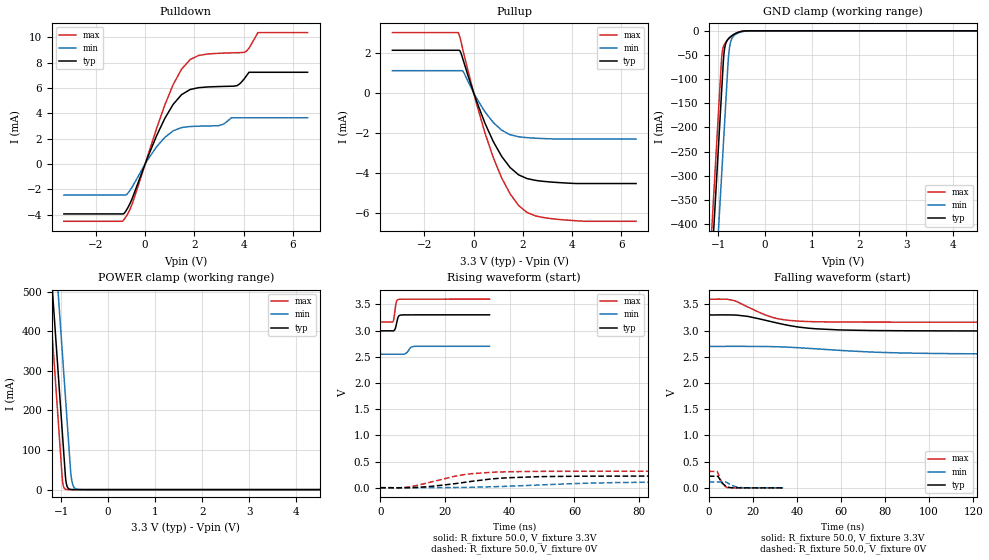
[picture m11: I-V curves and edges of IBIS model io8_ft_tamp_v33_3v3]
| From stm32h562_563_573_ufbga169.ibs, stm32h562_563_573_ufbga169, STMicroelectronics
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[Model]   io8_ft_tamp_v33_3v3
Model_type I/O
Polarity   Non-Inverting
Enable   Active-Low
| CAP_THRESHOLD on pad IOFT is "UDTCAPC" :
| Rising=20.0% of vddiom   Falling=80.0% of vddiom
| C_comp min and max val. don't necessarily correlate with the min and max pvt
| but are the smallest and greatest pad capacitance found.
| var   typ   min   max
C_comp   8.23612pF  8.16297pF  8.41737pF
|C_comp_pullup   5.18195pF  4.95450pF  4.90580pF
|C_comp_pulldown   3.05417pF  3.20847pF  3.51157pF
Vinl = 1.35V
Vinh = 1.8V
Vmeas = 1.65V   | Reference voltage for timing measurements
Cref  = 50.0pF   | Timing specification test load capacitance value
Rref  = 1.0MOhm   | Timing specification test load resistance value
Vref  = 1.815V   | Timing specification test load voltage
[Model Spec]
| TIME_THRESHOLD on pin ZIV33SW is "CMOS" :
| Rising=40.0% of VDDV33SW   Falling=60.0% of VDDV33SW
Vinl 1.28980V 1.06780V 1.39680V
Vinh 1.76120V 1.48020V 1.88320V
| variable   typ   min   max
[Temperature Range] 25.0 125.0 -40.0
| variable   typ   min   max
[Voltage Range] 3.3V 2.7V 3.6V
| variable   typ   min   max
[POWER Clamp Reference] 3.3V 2.7V 3.6V
| variable   typ   min   max
[GND Clamp Reference] 0V 0V 0V
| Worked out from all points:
|   slope of the pulldown table from 0 to 0.495 V, typ, clamps not added: 211 ohm
|   slope of the pullup table from 0 to 0.495 V, typ, clamps not added: 307 ohm
|   GND clamp passes 1 mA (typ) near -0.49 V on its own axis
|   POWER clamp passes 1 mA (typ) near -0.82 V on its own axis
|   rising waveform, R_fixture 50.0, V_fixture 3.3V: 20-80 % time 707ps typ, 1.09ns min, 576ps max; typ from 2.99 V to 3.3 V
|   falling waveform, R_fixture 50.0, V_fixture 3.3V: 20-80 % time 22.1ns typ, 40.6ns min, 14.5ns max; typ from 3.3 V to 2.99 V
|   rising waveform, R_fixture 50.0, V_fixture 0V: 20-80 % time 17.9ns typ, 30.6ns min, 13.5ns max; typ from 0 V to 0.222 V
|   falling waveform, R_fixture 50.0, V_fixture 0V: 20-80 % time 2.6ns typ, 3.54ns min, 2.19ns max; typ from 0.222 V to 0 V
[POWER Clamp]
-3.3V     4.099A     4.3A       3.98A
-1.25V    613.6mA    815.2mA    494.9mA
-1.17V    477.6mA    679.2mA    358.9mA
-1.13V    409.6mA    611.2mA    290.9mA
-1.02V    222.6mA    424.2mA    103.9mA
-970mV    137.6mA    339.2mA    21.83mA
-910mV    35.64mA    237.2mA    1.102mA
-870mV    7.512mA    169.2mA    150.4uA
-790mV    333.8uA    37.52mA    2.807uA
-750mV    70.36uA    11.69mA    384.4nA
-670mV    3.13uA     1.135mA    8.16nA
6.6V      0A         0A         0A
[GND Clamp]
-3.3V     -4.162A    -4.335A    -4.091A
-1.25V    -676.6mA   -850mA     -605.8mA
-930mV    -132.6mA   -306mA     -61.84mA
-910mV    -98.56mA   -272mA     -42.23mA
-880mV    -51.44mA   -221mA     -30.61mA
-860mV    -35.47mA   -187mA     -26.73mA
-790mV    -17.33mA   -67.97mA   -18.18mA
-770mV    -15.12mA   -44.17mA   -16.25mA
-740mV    -12.41mA   -25.47mA   -13.56mA
-710mV    -10.15mA   -16.48mA   -11.11mA
-580mV    -3.392mA   -4.732mA   -3.302mA
6.6V      12.65nA    2.523uA    1.261nA
| variable   typ   min   max
[Pullup Reference] 3.3V 2.7V 3.6V
| variable   typ   min   max
[Pulldown Reference] 0V 0V 0V
[Pullup]
-3.3V     2.116mA    1.098mA    2.998mA
-620mV    2.116mA    1.098mA    2.978mA
-540mV    2.045mA    1.098mA    2.681mA
-420mV    1.613mA    1.045mA    2.057mA
120mV     -423.9uA   -273uA     -554.9uA
800mV     -2.438mA   -1.486mA   -3.239mA
1.14V     -3.174mA   -1.869mA   -4.248mA
1.48V     -3.724mA   -2.094mA   -5.036mA
1.83V     -4.094mA   -2.195mA   -5.624mA
2.17V     -4.278mA   -2.239mA   -5.967mA
3.6V      -4.488mA   -2.312mA   -6.328mA
6.6V      -4.526mA   -2.312mA   -6.407mA
[Pulldown]
-3.3V     -3.928mA   -2.441mA   -4.51mA
-860mV    -3.894mA   -2.441mA   -4.374mA
-510mV    -2.641mA   -1.761mA   -3.058mA
800mV     3.6mA      2.103mA    4.66mA
1.48V     5.472mA    2.879mA    7.48mA
1.83V     5.88mA     2.962mA    8.24mA
2.99V     6.111mA    3.028mA    8.73mA
3.73V     6.183mA    3.65mA     8.778mA
4.05V     6.78mA     3.65mA     8.827mA
4.22V     7.236mA    3.65mA     9.137mA
4.58V     7.236mA    3.65mA     10.37mA
6.6V      7.236mA    3.65mA     10.37mA
[Ramp]
dV/dt_r 133.32367mV/17.7581ns 68.09984mV/29.89831ns 188.78372mV/13.46674ns
dV/dt_f 183.37714mV/21.73988ns 90.192mV/40.14624ns 262.38562mV/14.43737ns
R_load = 50.0
| Removed startup time: 0s 0s 0s  .
| Removed end time: 33.75ns.
[Rising Waveform]
R_fixture   = 50.0
V_fixture   = 3.3V
V_fixture_min = 2.7V
V_fixture_max = 3.6V
0s        2.994V     2.55V      3.163V
3.9ns     2.993V     2.55V      3.168V
4.25ns    3V         2.55V      3.238V
4.65ns    3.039V     2.55V      3.425V
4.95ns    3.108V     2.55V      3.539V
5.7ns     3.275V     2.55V      3.595V
7.6ns     3.299V     2.553V     3.599V
9.45ns    3.3V       2.678V     3.6V
10.35ns   3.3V       2.698V     3.6V
33.75ns   3.3V       2.7V       3.6V
| Removed startup time: 0s 0s 0s  .
| Removed end time: 598.75ns.
[Falling Waveform]
R_fixture   = 50.0
V_fixture   = 3.3V
V_fixture_min = 2.7V
V_fixture_max = 3.6V
0s        3.3V       2.7V       3.6V
8.1ns     3.301V     2.701V     3.601V
11.2ns    3.3V       2.701V     3.578V
23.8ns    3.217V     2.699V     3.333V
31.2ns    3.145V     2.693V     3.23V
40.7ns    3.069V     2.675V     3.182V
48.9ns    3.035V     2.653V     3.17V
85.55ns   2.999V     2.577V     3.163V
134.4ns   2.995V     2.555V     3.163V
598.7ns   2.994V     2.55V      3.163V
| Removed startup time: 0s 0s 0s  .
| Removed end time: 598.6ns.
[Rising Waveform]
R_fixture   = 50.0
V_fixture   = 0V
V_fixture_min = 0V
V_fixture_max = 0V
0s        187.9nV    1.752uV    236.8nV
5ns       -2.009mV   2.578uV    -2.772mV
9.3ns     1.489mV    -1.245mV   17.7mV
22.6ns    73.66mV    3.679mV    212.1mV
28.2ns    121.4mV    8.332mV    267.1mV
36.7ns    179.2mV    21.97mV    299.8mV
48.9ns    210.6mV    51.52mV    311.7mV
73.3ns    221.3mV    98.2mV     314.4mV
110ns     222.1mV    112mV      314.6mV
598.6ns   222.2mV    113.5mV    314.6mV
| Removed startup time: 0s 0s 0s  .
| Removed end time: 33.75ns.
[Falling Waveform]
R_fixture   = 50.0
V_fixture   = 0V
V_fixture_min = 0V
V_fixture_max = 0V
0s        222.2mV    113.5mV    314.6mV
3.75ns    222.3mV    113.5mV    314mV
4.35ns    209.1mV    113.5mV    264.2mV
5.1ns     156.4mV    113.5mV    178mV
6.2ns     89.56mV    113.5mV    89.74mV
7.05ns    56.09mV    113.5mV    43mV
8.3ns     22.28mV    101.8mV    8.598mV
11.05ns   1.361mV    36.31mV    784.7uV
14.5ns    321.2uV    6.504mV    218.7uV
33.75ns   53.43uV    57.58uV    51.85uV
